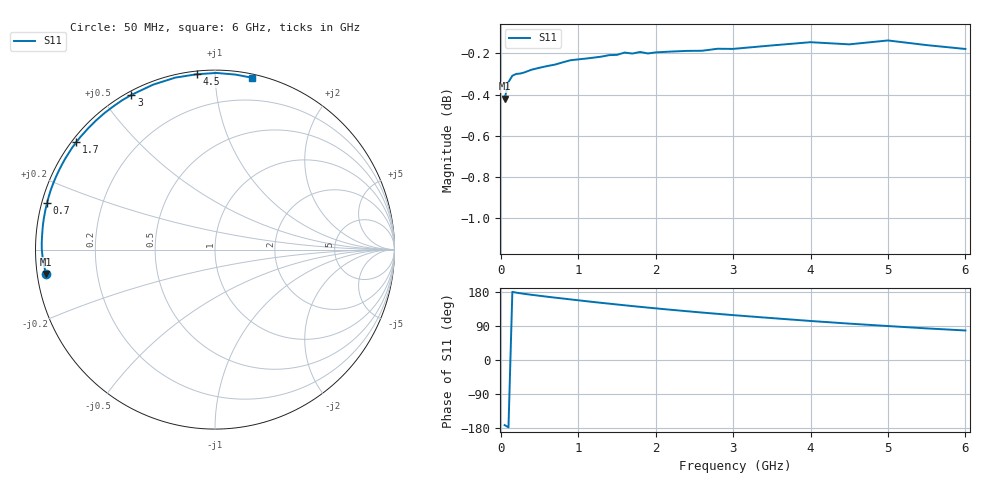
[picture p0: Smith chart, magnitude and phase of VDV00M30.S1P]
! Infineon Technologies  Discrete & RF Semiconductors
! BBY 55-03
! Si Tuning Diode in SOD323
! VR =
! S-Parameters:  June  1999
# GHz  S  MA  R  50
!  f  S11
! GHz  MAG  ANG
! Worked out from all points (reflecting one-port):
!   34 points, 50 MHz to 6 GHz, reference 50 ohm
!   lowest |S11| = -0.4 dB at 50 MHz (marker M1), VSWR 41.35, Z = 1.22 - j3.58 ohm
!   phase of S11 starts at -172 deg and turns -110 deg over the sweep
!   S11 on the Smith chart (normalised r, x): 50 MHz: 0.02, -0.07; 700 MHz: 0.01, +0.14; 1.7 GHz: 0.01, +0.34; 3 GHz: 0.01, +0.60; 4.5 GHz: 0.02, +0.90; 6 GHz: 0.03, +1.24
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0.05  0.9528 -171.8
0.1  0.9617 -177.6
0.15  0.9651 179.8
0.2  0.9661 177.8
0.3  0.9668 174.7
0.4  0.9684 172.0
0.5  0.9694 169.5
0.7  0.9711 164.6
0.8  0.9724 162.3
0.9  0.9735 159.9
1  0.974 157.6
1.2  0.9749 153.0
1.4  0.9763 148.7
1.6  0.9777 144.4
1.7  0.9771 142.3
1.8  0.978 140.3
2  0.9778 136.3
2.2  0.9782 132.5
2.4  0.9786 128.8
2.6  0.9787 125.2
2.8  0.9798 121.8
3  0.9797 118.4
3.5  0.9816 110.6
4  0.9834 103.0
4.5  0.9822 96.0
5  0.9843 89.6
5.5  0.9818 83.4
6  0.9797 77.9
